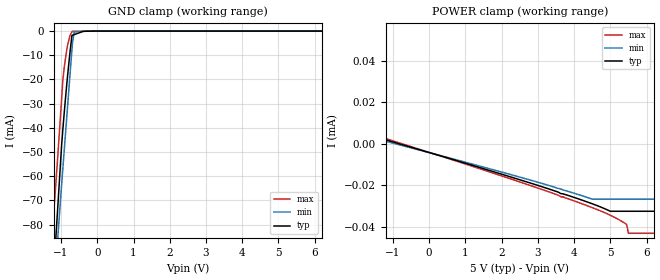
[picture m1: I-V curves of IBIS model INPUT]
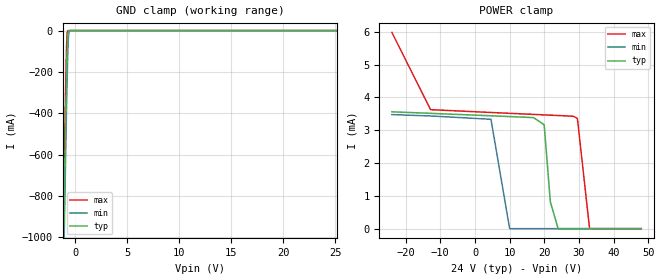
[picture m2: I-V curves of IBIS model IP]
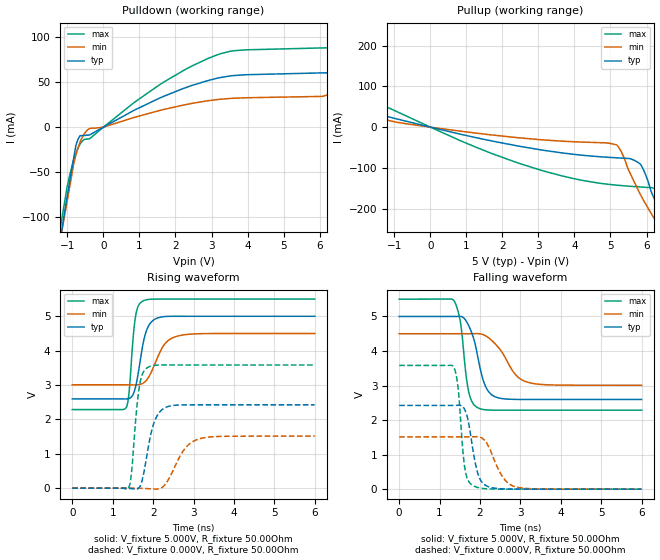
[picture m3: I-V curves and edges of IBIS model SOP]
|Texas Instruments Incorporated
|Industrial 8-Digital-Input Serializer
| Marketing part#   Voltage Range   Package-type   #pins/pkg drawing
|SN65HVS882PWP   4.5V to 5.5V   HTSSOP   28pin-PWP
|SN65HVS882PWPG4   4.5V to 5.5V   HTSSOP   28pin-PWP
|SN65HVS882PWPR   4.5V to 5.5V   HTSSOP   28pin-PWP
|SN65HVS882PWPRG4   4.5V to 5.5V   HTSSOP   28pin-PWP
[IBIS Ver]   4.0
[File name]   sn65hvs882.ibs
[File Rev]   2.0
[Date]   10/01/2008
[Source]   Texas Instruments Incorporated.
   Analog-eLab, HPA
   12500 TI Blvd
   Dallas, TX -75243
   For Support e-mail: elab_ibis@list.ti.com  OR
   Contact Texas Instruments at ATTN:DATA TRANSMISSIONS
[Notes]   Revision History:
   2.0: 10/01/2008
   - Buffer characteristics not matched to measurements
   - ccomp correlated to measurements
   - IBIS correlated to TISPICE
[Disclaimer]
(C) Copyright Texas Instruments Incorporated 2008
   All rights reserved
  Texas Instruments Incorporated hereby grants the user of this IBIS
model a non-exclusive, nontransferable license to use this IBIS model
under the following terms.  Before using this IBIS model, the user
should read this license.  If the user does not accept these terms,
the IBIS model should be returned to Texas Instruments within 30 days.
  The user is granted this license only to use the IBIS model and
is not granted rights to sell, load, rent, lease or license the IBIS
model in whole or in part, or in modified form to anyone other than
user.  User may modify the IBIS model to suit its specific applications
but rights to derivative works and such modifications shall belong to
Texas Instruments.
  This IBIS model is provided on an "AS IS" basis and Texas Instruments
makes absolutely no warranty with respect to the information contained
herein.  TEXAS INSTRUMENTS DISCLAIMS AND CUSTOMER WAIVES ALL WARRANTIES,
EXPRESS OR IMPLIED, INCLUDING WARRANTIES OF MERCHANTABILITY OR FITNESS
FOR A PARTICULAR PURPOSE. The entire risk as to quality and performance
is with the Customer. ACCORDINGLY, IN NO EVENT SHALL THE COMPANY BE LIABLE
FOR ANY DAMAGES, WHETHER IN CONTRACT OR TORT,INCLUDING ANY LOST PROFITS
OR OTHER INCIDENTAL, CONSEQUENTIAL, EXEMPLARY, OR PUNITIVE DAMAGES ARISING
OUT OF THE USE OR APPLICATION OF THE IBIS model provided in this package.
Further, Texas Instruments reserves the right to discontinue or make changes
without notice to any product herein to improve reliability, function, or
design. Texas Instruments does not convey any license under patent rights
or any other intellectual property rights, including those of third parties.
[Copyright]   Copyright 2008, Texas Instruments, All Rights Reserved
[Component]   SN65HVS882
[Manufacturer]  Texas Instruments Incorporated
[Package]
|   typ   min   max
R_pkg   0.140   0.092   0.189
L_pkg   3.232nH   2.159nH   4.305nH
C_pkg   0.546pF   0.424pF   0.668pF
[Pin]   signal_name   model_name   R_pin   L_pin   C_pin
1   DB0   INPUT   0.18872  4.30519nH  0.61875pF
2   DB1   INPUT   0.18688  3.91193nH  0.58027pF
3   IP0   IP   0.17609  3.44027nH  0.49863pF
4   RE0   NC   0.14456  2.95170nH  0.48588pF
5   IP1   IP   0.12099  2.58952nH  0.46045pF
6   RE1   NC   0.10280  2.31882nH  0.43775pF
7   IP2   IP   0.09328  2.17530nH  0.42758pF
8   RE2   NC   0.09329  2.17726nH  0.42772pF
9   IP3   IP   0.10286  2.32875nH  0.44084pF
10   RE3   NC   0.12103  2.59710nH  0.46070pF
11   IP4   IP   0.14461  2.96063nH  0.48587pF
12   RE4   NC   0.17614  3.45066nH  0.49636pF
13   RLIM   NC   0.16787  3.62755nH  0.56131pF
14   VCC   POWER   0.09356  3.59739nH  0.64831pF
15   5VOP   NC   0.08817  3.44134nH  0.63929pF
16   TOK   NC   0.19409  4.03351nH  0.59029pF
17   RE5   NC   0.17614  3.45069nH  0.50197pF
18   IP5   IP   0.14460  2.96053nH  0.48642pF
19   RE6   NC   0.12103  2.59712nH  0.46073pF
20   IP6   IP   0.10286  2.32876nH  0.44079pF
21   RE7   NC   0.09330  2.17752nH  0.42741pF
22   IP7   IP   0.09328  2.17532nH  0.42443pF
23   SOP   SOP   0.09210  2.15895nH  0.42517pF
24   CEB   INPUT   0.10191  2.29956nH  0.44266pF
25   CLK   INPUT   0.12407  2.63619nH  0.46625pF
26   LDB   INPUT   0.15544  3.11954nH  0.48079pF
27   SIP   INPUT   0.18683  3.90932nH  0.57801pF
28   GND   GND   0.10599  3.90252nH  0.66748pF
| Models and submodels in the file (3): INPUT (Input), IP (Input), SOP (Output)
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|   INPUT MODEL
[Model]   INPUT
Model_type   Input
|Signals   CLK,LDB,SIP,CEB,DB0,DB1
|Input Levels
Vinl = 0.4V   |not specified used avg of corner cases
Vinh = 3.75V   |not specified used avg of corner cases
|   typ   min   max
C_comp   1.82pF   1.74pF   1.90pF
[Model Spec]
| Input levels across the corners
|   typ   min   max
Vinl   0.4V   0.0V   0.8V
Vinh   3.75V   2.0V   5.5V
[Voltage Range]   5.0V   4.5V   5.5V
[Power Clamp Reference]   5.0V   4.5V   5.5V
| Junction Temperature (Ambient temp is 15C typ, 85C min,  -40C max)
[Temperature Range]   27.0   100.0   -40.0
[GND Clamp]
|   Voltage   I(typ)   I(min)   I(max)
-5V       -525.1mA   -514.5mA   -492.8mA
-1.25V    -109.3mA   -116.5mA   -84.72mA
-1.183V   -94.35mA   -103.8mA   -71.28mA
-1.15V    -86.69mA   -97.24mA   -64.36mA
-1.1V     -74.98mA   -87.28mA   -53.74mA
-983.3mV  -46.88mA   -63.27mA   -27.81mA
-950mV    -40.55mA   -56.7mA    -20.1mA
-883.3mV  -28.71mA   -43.58mA   -11.74mA
-816.7mV  -17.96mA   -30.48mA   -5.651mA
-700mV    -1.773mA   -7.619mA   -290.2uA
-383.3mV  -106.9uA   -73.78uA   NA
9.983V    0A         0A         0A
[POWER Clamp]
|   Voltage   I(typ)   I(min)   I(max)
-5V       284.9uA    283.6uA    283.6uA
-4.983V   21.61uA    18.86uA    23.95uA
-4.967V   20.98uA    18.26uA    23.34uA
816.7mV   -8.358uA   -7.962uA   -8.662uA
3.633V    -23.97uA   -21.79uA   -25.46uA
3.717V    -24.22uA   -22.3uA    -25.55uA
4.5V      -28.87uA   -26.65uA   -30.73uA
5V        -32.49uA   -26.65uA   -34.4uA
5.2V      -32.49uA   -26.65uA   -36.17uA
5.45V     -32.49uA   -26.65uA   -38.8uA
5.5V      -32.49uA   -26.65uA   -43.12uA
9.983V    -32.49uA   -26.65uA   -43.12uA
|   IP MODEL
[Model]   IP
Model_type   Input
|Signals   IPx [x = 0 to 7]
|Hysterisis parameters
|Input Levels
Vinl = 2.0V
Vinh = 19.75V
|   typ   min   max
C_comp   7.61pF   7.22pF   7.64pF
[Model Spec]
| Input levels across the corners
|   typ   min   max
Vinl   2.0V   0.0V   4.0V
Vinh   19.75V   5.5V   34V
| Hysterisis Input levels
Vinh+   9.4V   NA   10V
Vinh-   8.4V   6.0V   NA
Vinl+   5.2V   NA   5.5V
Vinl-   4.3V   4.0V   NA
[Voltage Range]   24.0V   10V   34V
[Pullup Reference]   24.0V   10V   34V
[Power Clamp Reference]   24.0V   10V   34V
| Junction Temperature (Ambient temp is 15C typ, 85C min,  -40C max)
[Temperature Range]   27.0   100.0   -40.0
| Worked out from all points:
|   GND clamp passes 1 mA (typ) near -0.62 V on its own axis
[GND Clamp]
|   Voltage   I(typ)   I(min)   I(max)
-24V      -74.15A    -74.42A    -73.8A
-1.165V   -1.145A    -1.299A    -971.1mA
-1.12V    -1.01A     -1.165A    -836.2mA
-1.08V    -891.8mA   -1.047A    -717.6mA
-1.04V    -774.6mA   -930.2mA   -600.7mA
-855mV    -268.5mA   -417mA     -116mA
-790mV    -124.8mA   -257.9mA   -21.13mA
-740mV    -47.14mA   -152.4mA   -2.515mA
-695mV    -12.94mA   -78.07mA   -305uA
-610mV    -635.6uA   -11.13mA   -7.078uA
-460mV    -3.809uA   -148.5uA   -1.702uA
48V       0A         0A         0A
[POWER Clamp]
| IPNEW_34
|   Voltage   I(typ)   I(min)   I(max)
-24V      3.564mA    3.479mA    5.985mA
-12.84V   3.517mA    3.436mA    3.629mA
4.605V    3.442mA    3.336mA    3.543mA
10.45V    3.416mA    NA         3.515mA
16.93V    3.386mA    NA         3.485mA
19.97V    3.167mA    NA         3.47mA
21.75V    820.5uA    NA         3.461mA
24V       0A         NA         NA
34V       0A         0A         0A
48V       0A         0A         0A
|   SOP Model
[Model]   SOP
Model_type   Output
| Signals   SOP
Cref = 10pF   |Timing specification test load capacitance value
Rref = 0.00Ohm
| variable   typ   min   max
C_comp   3.56pF   3.48pF   3.64pF
[Model Spec]
|Timing spec test load voltage corners 0.45*VCC
Vmeas   2.5V   2.25V   2.75V
|Vref   2.5V   2.25V   2.75V
| Junction Temperature (Ambient temp is 15C typ, 85C min,  -40C max)
[Temperature Range]   27.0   100.0   -40.0
[Voltage range]   5.0V   4.5V   5.5V
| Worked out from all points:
|   slope of the pulldown table from 0 to 0.75 V, typ, clamps not added: 45.5 ohm
|   slope of the pullup table from 0 to 0.75 V, typ, clamps not added: 48.1 ohm
|   falling waveform, V_fixture 5.000V, R_fixture 50.00Ohm: 20-80 % time 304ps typ, 509ps min, 188ps max; typ from 5 V to 2.6 V
|   rising waveform, V_fixture 5.000V, R_fixture 50.00Ohm: 20-80 % time 228ps typ, 370ps min, 133ps max; typ from 2.6 V to 5 V
|   rising waveform, V_fixture 0.000V, R_fixture 50.00Ohm: 20-80 % time 258ps typ, 428ps min, 161ps max; typ from 0 V to 2.42 V
|   falling waveform, V_fixture 0.000V, R_fixture 50.00Ohm: 20-80 % time 225ps typ, 370ps min, 148ps max; typ from 2.42 V to 0 V
[Pulldown]
|   Voltage   I(typ)   I(min)   I(max)
-5V       -739.4mA   -652.6mA   -844.4mA
-1.249V   -137.8mA   -136.4mA   -125mA
-1.039V   -84.91mA   -90.05mA   -74.12mA
-739.1mV  -17.27mA   -27.42mA   -26.62mA
-439.1mV  -8.866mA   -3.019mA   -13.11mA
1.541V    31.93mA    18.3mA     46.58mA
3.132V    54.07mA    30.49mA    79.88mA
6.192V    60.3mA     35.46mA    88.03mA
7.032V    66.82mA    58.88mA    88.82mA
7.362V    82.94mA    69.23mA    90.11mA
7.813V    106.3mA    83.49mA    121.2mA
9.973V    221.3mA    152.7mA    308.9mA
[Pullup]
|   Voltage   I(typ)   I(min)   I(max)
-5V       227.3mA    142.3mA    359.5mA
-4.79V    211.3mA    130.6mA    336.5mA
-2.51V    89.56mA    57.58mA    137.9mA
-1.699V   47.48mA    32.2mA     72.03mA
-1.279V   28.78mA    19.82mA    52.28mA
2.351V    -44.92mA   -25.19mA   -85.36mA
5.172V    -75.25mA   -43.57mA   -142.3mA
5.832V    -90.96mA   -165.6mA   -146.8mA
6.312V    -194mA     -238.2mA   -157.3mA
6.642V    -250.2mA   -288.2mA   -205.8mA
6.822V    -277.5mA   -316.3mA   -247.2mA
9.973V    -796.1mA   -759.9mA   -792.8mA
[Ramp]
R_load = 50.00Ohm
|   typ   min   max
dV/dt_r   1.455V/257.028ps 907.647mV/427.286ps   2.149V/161.166ps
dV/dt_f   1.442V/303.841ps 895.762mV/508.627ps   1.928V/188.231ps
[Falling Waveform]
V_fixture = 5.000V
V_fixture_min = 4.500V
V_fixture_max = 5.500V
R_fixture = 50.00Ohm
|   Time   V(typ)   V(min)   V(max)
0s        4.999V     4.5V       5.499V
1.355ns   4.999V     4.499V     5.458V
1.515ns   5.001V     4.499V     4.848V
1.65ns    4.883V     4.499V     3.35V
1.725ns   4.723V     4.499V     2.797V
1.975ns   3.663V     4.499V     2.341V
2.12ns    3.023V     4.451V     2.299V
2.3ns     2.722V     4.294V     2.287V
3.165ns   2.596V     3.1V       2.286V
6ns       2.596V     3.007V     2.286V
[Rising Waveform]
V_fixture = 5.000V
V_fixture_min = 4.500V
V_fixture_max = 5.500V
R_fixture = 50.00Ohm
|   Time   V(typ)   V(min)   V(max)
0s        2.596V     3.007V     2.286V
1.34ns    2.595V     3.006V     2.351V
1.405ns   2.61V      3.005V     2.785V
1.51ns    2.739V     3.001V     4.43V
1.565ns   2.941V     3.002V     4.988V
1.765ns   4.279V     3.065V     5.453V
2.025ns   4.901V     3.564V     5.499V
2.285ns   4.991V     4.188V     5.5V
2.6ns     5V         4.422V     5.499V
6ns       4.999V     4.5V       5.499V
[Rising Waveform]
V_fixture = 0.000V
V_fixture_min = 0.000V
V_fixture_max = 0.000V
R_fixture = 50.00Ohm
|   Time   V(typ)   V(min)   V(max)
0s        -18.06uV   243uV      393.5uV
1.385ns   -3.823mV   768.5uV    -5.909mV
1.465ns   -12.66mV   930.2uV    441mV
1.585ns   -27.04mV   -336.7uV   2.2V
1.665ns   33.23mV    -2.473mV   2.993V
1.895ns   1.284V     -15.1mV    3.529V
2.215ns   2.277V     17.37mV    3.583V
2.785ns   2.423V     1.148V     3.582V
3.15ns    2.424V     1.437V     3.582V
6ns       2.424V     1.513V     3.582V
[Falling Waveform]
V_fixture = 0.000V
V_fixture_min = 0.000V
V_fixture_max = 0.000V
R_fixture = 50.00Ohm
|   Time   V(typ)   V(min)   V(max)
0s        2.424V     1.513V     3.582V
1.345ns   2.424V     1.513V     3.545V
1.46ns    2.428V     1.513V     2.914V
1.63ns    2.285V     1.514V     573.9mV
1.845ns   999.3mV    1.518V     91.15mV
1.97ns    375.7mV    1.511V     41.24mV
2.1ns     139.8mV    1.431V     17.17mV
2.54ns    11.08mV    391.4mV    1.21mV
2.86ns    1.785mV    74.72mV    573.2uV
6ns       -18.06uV   243uV      393.5uV
